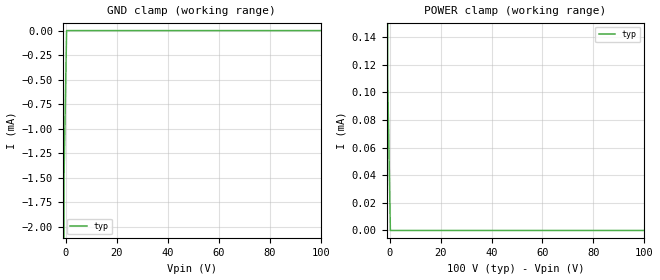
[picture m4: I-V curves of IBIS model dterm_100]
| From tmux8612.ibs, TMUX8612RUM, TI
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| dterm_100
[Model]   dterm_100
Model_type   Terminator
|   typ   min   max
C_comp   1.008417e-11   NA   NA
[Voltage Range]   100   NA   NA
[Temperature Range]   27   NA   NA
[Power Clamp Reference]   100   NA   NA
[GND Clamp Reference]   0   NA   NA
[GND Clamp]
|   Voltage   I(typ)   I(min)   I(max)
-5V       -2.409A    NA         NA
-1.818V   -287mA     NA         NA
-757.6mV  -1.566mA   NA         NA
303mV     -1.198nA   NA         NA
100V      2.96nA     NA         NA
[POWER Clamp]
|   Voltage   I(typ)   I(min)   I(max)
-5V       1.055A     NA         NA
-1.818V   191.2mA    NA         NA
-758mV    111.3uA    NA         NA
303mV     2.957nA    NA         NA
100V      -1.21nA    NA         NA
